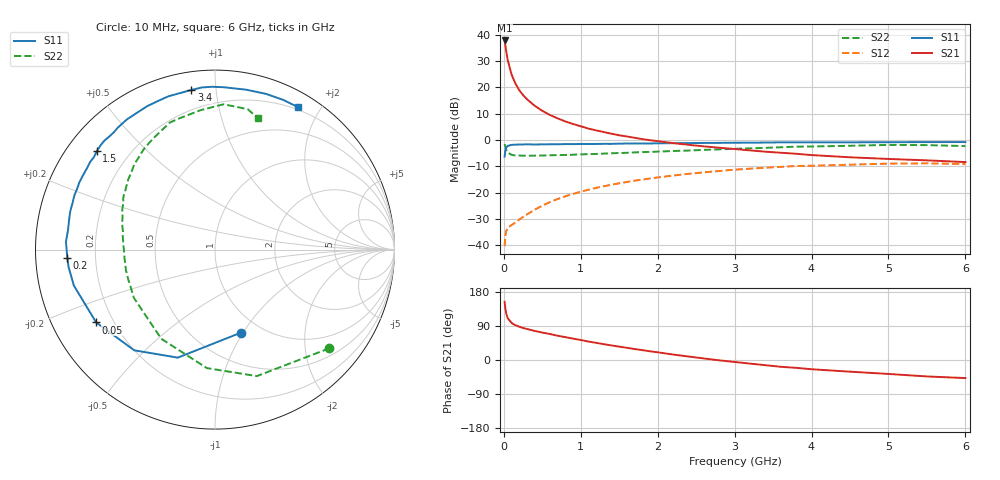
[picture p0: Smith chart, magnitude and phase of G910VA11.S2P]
! SIEMENS Small Signal Semiconductors
! BFG235
! Si NPN RF Bipolar Junction Transistor in SOT223
! VCE = 10 V  IC = 110 mA
! Common Emitter S-Parameters:  July  1994
# GHz  S  MA  R  50
!  f  S11  S21  S12  S22
! GHz  MAG  ANG  MAG  ANG  MAG  ANG  MAG  ANG
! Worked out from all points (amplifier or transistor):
!   40 points, 10 MHz to 6 GHz, reference 50 ohm
!   highest |S21| = 37.8 dB at 10 MHz (marker M1)
!   |S21| within 3 dB of that: start of sweep to 25.24 MHz
!   unconditionally stable (mu >= 1): 475.4 MHz to 1.484 GHz
!   at 200 MHz: K = 0.76, MSG = 24.6 dB, |S12| = -30.2 dB
!   at 1.5 GHz: K = 1.00, MSG = 9.1 dB, |S12| = -16.4 dB
!   at 6 GHz: K = 0.90, MSG = 0.4 dB, |S12| = -9.1 dB
!   S11 on the Smith chart (normalised r, x): 10 MHz: 0.81, -0.98; 50 MHz: 0.14, -0.28; 200 MHz: 0.10, -0.03; 1.5 GHz: 0.09, +0.36; 3.4 GHz: 0.09, +0.86; 6 GHz: 0.17, +1.73
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0.01  0.4848 -72.6  77.96 153.7  0.0097 63.9  0.8415 -40.8
0.02  0.6366 -109.0  62.31 135.2  0.0154 49.9  0.7424 -71.7
0.03  0.7192 -128.7  49.42 123.4  0.0186 41.8  0.6619 -93.9
0.05  0.7766 -148.5  33.25 110.4  0.0215 33.8  0.5799 -121.1
0.1  0.8115 -165.7  17.66 97.9  0.0244 34.6  0.5259 -149.1
0.15  0.8213 -173.1  11.88 91.8  0.0272 40.1  0.5112 -160.8
0.2  0.8242 -176.9  8.902 87.8  0.031 44.8  0.5093 -167.1
0.25  0.8269 179.7  7.166 84.5  0.0348 48.7  0.506 -171.3
0.3  0.8316 177.1  5.985 81.9  0.0388 51.8  0.5066 -174.6
0.4  0.8261 172.3  4.503 76.8  0.0476 55.7  0.5069 -179.1
0.5  0.8296 168.4  3.595 72.4  0.057 57.4  0.5106 177.4
0.6  0.8341 165.3  3 68.5  0.0666 58.5  0.5149 174.3
0.7  0.8353 161.7  2.584 64.0  0.0763 58.7  0.5196 171.5
0.9  0.8396 156.2  2.023 56.4  0.0951 57.4  0.5285 167.0
1.1  0.844 149.9  1.656 48.6  0.1144 55.4  0.5414 162.5
1.5  0.8567 140.3  1.234 35.3  0.1516 49.5  0.5691 154.4
2.2  0.8758 124.1  0.879 14.4  0.2122 37.3  0.6215 141.1
3.2  0.8934 102.7  0.638 -9.5  0.287 18.0  0.698 121.9
3.4  0.8994 98.4  0.603 -13.7  0.2989 14.0  0.7139 117.6
4.5  0.9077 78.9  0.472 -30.8  0.3413 -7.2  0.7808 96.0
5.5  0.9165 65.6  0.413 -43.4  0.3622 -25.8  0.8034 76.9
6  0.9186 59.8  0.383 -47.7  0.3517 -32.7  0.7699 71.9
